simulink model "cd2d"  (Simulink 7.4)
settings: Solver=ode45  StartTime=0.0  StopTime=10.0  RelTol=1e-3
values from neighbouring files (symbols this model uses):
  B = 8    [cd2d_par.m]
  D = 5    [cd2d_par.m]
  T = 12    [cd2d_par.m]
libraries: simulink x2

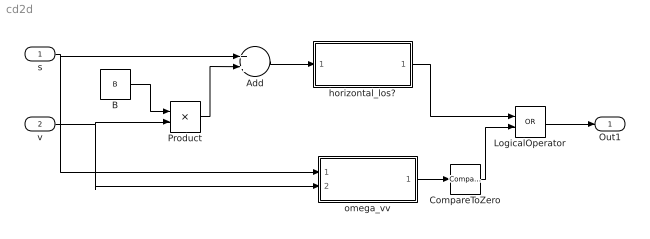
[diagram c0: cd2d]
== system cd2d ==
  s : Inport  Description=|  OutDataType=fixdt(1, 16)  OutScaling=2^0
      | begin dimension                   
      | output _ : [(length kilometer 1)];
      | end dimension
  v : Inport  Description=|  Port=2  OutDataType=fixdt(1, 16)  OutScaling=2^0
      | begin dimension                                 
      | output _ : [(length kilometer 1, time hour -1)];
      | end dimension
  Add : Sum  OutDataType=fixdt(1, 16)  OutScaling=2^-10
  B : Constant  Description=|  Value=B  OutDataType=fixdt(1, 16)  OutScaling=2^0
      | begin dimension            
      | output _ : [(time hour 1)];
      | end dimension
  CompareToZero : simulink/Logic and Bit Operations/Compare To Zero  SystemSampleTime=-1  relop=<  LogicOutDataTypeMode=uint8
  LogicalOperator : Logic  Operator=OR  AllPortsSameDT=off  OutDataTypeMode=boolean  LogicDataType=fixdt(0, 8)  OutDataTypeStr=boolean
  Product : Product  OutDataType=fixdt(1, 16)  OutScaling=2^0
  horizontal_los? : Subsystem
  omega_vv : Subsystem
  Out1 : Outport  Description=|  OutDataType=fixdt(1, 16)  OutScaling=2^0
      | begin dimension             
      | input _ : [(dimensionless)];
      | end dimension
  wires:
  s/1 -> Add/1, omega_vv/1(s)
  B/1 -> Product/1
  v/1 -> Product/2, omega_vv/2(v)
  Product/1 -> Add/2
  Add/1 -> horizontal_los?/1(In1)
  horizontal_los?/1(Out1) -> LogicalOperator/1
  omega_vv/1(Out1) -> CompareToZero/1
  CompareToZero/1 -> LogicalOperator/2
  LogicalOperator/1 -> Out1/1

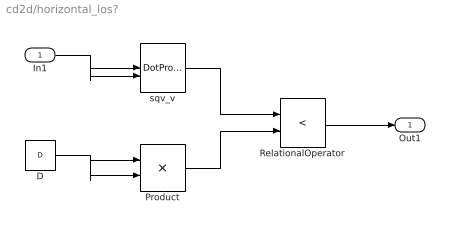
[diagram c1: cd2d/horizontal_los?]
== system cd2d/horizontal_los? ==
  In1 : Inport  Description=|  OutDataType=fixdt(1, 16)  OutScaling=2^0
      | begin dimension                   
      | output _ : [(length kilometer 1)];
      | end dimension
  D : Constant  Description=|  Value=D  OutDataType=fixdt(1, 16)  OutScaling=2^0
      | begin dimension                   
      | output _ : [(length kilometer 1)];
      | end dimension
  Product : Product  OutDataType=fixdt(1, 16)  OutScaling=2^0
  RelationalOperator : RelationalOperator  Operator=<  LogicOutDataTypeMode=boolean  LogicDataType=fixdt(0, 8)  OutDataTypeStr=boolean
  sqv_v : DotProduct  OutDataType=fixdt(1, 16)  OutScaling=2^-10
  Out1 : Outport  Description=|  OutDataType=fixdt(1, 16)  OutScaling=2^0
      | begin dimension             
      | input _ : [(dimensionless)];
      | end dimension
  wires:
  In1/1 -> sqv_v/1, sqv_v/2
  sqv_v/1 -> RelationalOperator/1
  Product/1 -> RelationalOperator/2
  RelationalOperator/1 -> Out1/1
  D/1 -> Product/1, Product/2

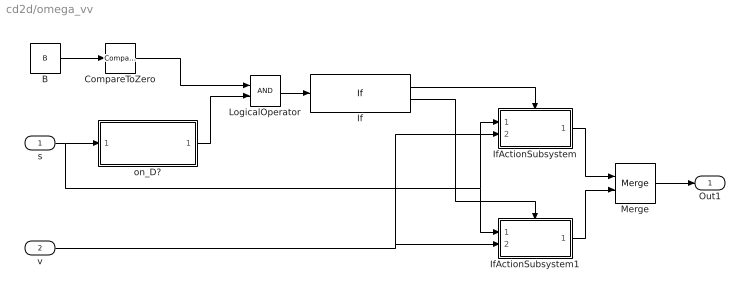
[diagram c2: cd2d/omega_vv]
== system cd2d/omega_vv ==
  s : Inport  Description=|  OutDataType=fixdt(1, 16)  OutScaling=2^0
      | begin dimension                   
      | output _ : [(length kilometer 1)];
      | end dimension
  v : Inport  Description=|  Port=2  OutDataType=fixdt(1, 16)  OutScaling=2^0
      | begin dimension                                 
      | output _ : [(length kilometer 1, time hour -1)];
      | end dimension
  B : Constant  Description=|  Value=B  OutDataType=fixdt(1, 16)  OutScaling=2^0
      | begin dimension            
      | output _ : [(time hour 1)];
      | end dimension
  CompareToZero : simulink/Logic and Bit Operations/Compare To Zero  SystemSampleTime=-1  relop===  LogicOutDataTypeMode=uint8
  If : If  IfExpression=u1
  IfActionSubsystem : Subsystem  TreatAsAtomicUnit=on
  IfActionSubsystem1 : Subsystem  TreatAsAtomicUnit=on
  LogicalOperator : Logic  AllPortsSameDT=off  OutDataTypeMode=boolean  LogicDataType=fixdt(0, 8)  OutDataTypeStr=boolean
  Merge : Merge
  on_D? : Subsystem
  Out1 : Outport  OutDataType=fixdt(1, 16)  OutScaling=2^0
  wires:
  s/1 -> IfActionSubsystem/1(s), IfActionSubsystem1/1(s), on_D?/1(In1)
  B/1 -> CompareToZero/1
  CompareToZero/1 -> LogicalOperator/1
  on_D?/1(Out1) -> LogicalOperator/2
  LogicalOperator/1 -> If/1
  Merge/1 -> Out1/1
  IfActionSubsystem/1(Out1) -> Merge/1
  IfActionSubsystem1/1(Out1) -> Merge/2
  If/2 -> IfActionSubsystem1/Action
  If/1 -> IfActionSubsystem/Action
  v/1 -> IfActionSubsystem/2(v), IfActionSubsystem1/2(v)

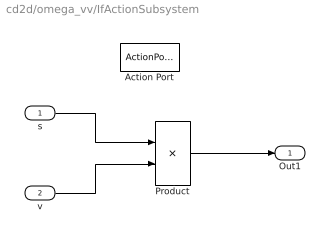
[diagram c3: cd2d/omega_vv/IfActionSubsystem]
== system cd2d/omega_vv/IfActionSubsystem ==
  s : Inport  Description=|  OutDataType=fixdt(1, 16)  OutScaling=2^0
      | begin dimension                   
      | output _ : [(length kilometer 1)];
      | end dimension
  v : Inport  Description=|  Port=2  OutDataType=fixdt(1, 16)  OutScaling=2^0
      | begin dimension                                 
      | output _ : [(length kilometer 1, time hour -1)];
      | end dimension
  Action Port : ActionPort  ActionType=then
  Product : Product  OutDataType=fixdt(1, 16)  OutScaling=2^0
  Out1 : Outport  Description=|  OutDataType=fixdt(1, 16)  OutScaling=2^0
      | begin dimension                                
      | input _ : [(length kilometer 2, time hour -1)];
      | end dimension
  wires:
  Product/1 -> Out1/1
  s/1 -> Product/1
  v/1 -> Product/2

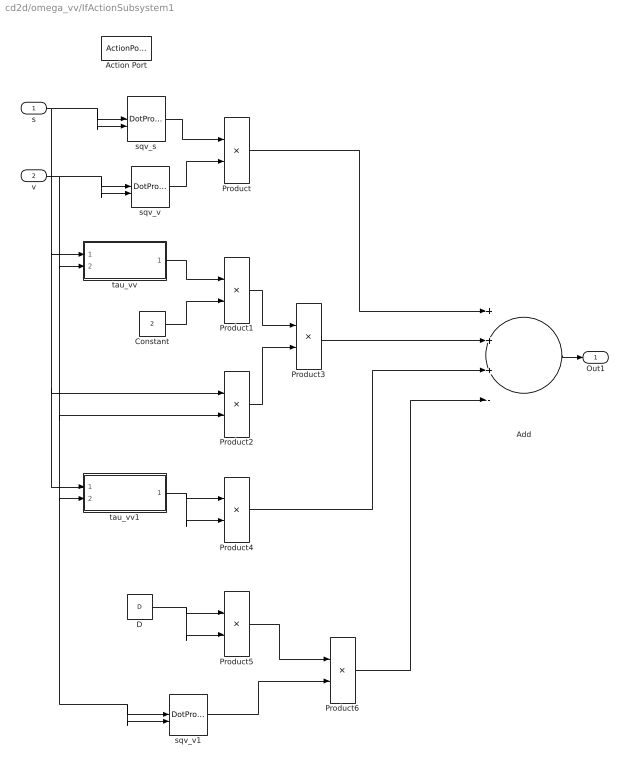
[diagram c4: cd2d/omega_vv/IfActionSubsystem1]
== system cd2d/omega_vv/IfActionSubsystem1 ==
  s : Inport  Description=|  OutDataType=fixdt(1, 16)  OutScaling=2^0
      | begin dimension                   
      | output _ : [(length kilometer 1)];
      | end dimension
  v : Inport  Description=|  Port=2  OutDataType=fixdt(1, 16)  OutScaling=2^0
      | begin dimension                                 
      | output _ : [(length kilometer 1, time hour -1)];
      | end dimension
  Action Port : ActionPort  ActionType=else
  Add : Sum  Inputs=+++-  OutDataType=fixdt(1, 16)  OutScaling=2^-10
  Constant : Constant  Description=|  Value=2  OutDataType=fixdt(1, 16)  OutScaling=2^0
      | begin dimension              
      | output _ : [(dimensionless)];
      | end dimension
  D : Constant  Description=|  Value=D  OutDataType=fixdt(1, 16)  OutScaling=2^0
      | begin dimension                   
      | output _ : [(length kilometer 1)];
      | end dimension
  Product{,1..6} (7 alike) : Product  OutDataType=fixdt(1, 16)  OutScaling=2^0
  sqv_s : DotProduct  OutDataType=fixdt(1, 16)  OutScaling=2^-10
  sqv_v : DotProduct  OutDataType=fixdt(1, 16)  OutScaling=2^-10
  sqv_v1 : DotProduct  OutDataType=fixdt(1, 16)  OutScaling=2^-10
  tau_vv : Subsystem
  tau_vv1 : Subsystem
  Out1 : Outport  Description=|  OutDataType=fixdt(1, 16)  OutScaling=2^0
      | begin dimension                                
      | input _ : [(length kilometer 4, time hour -2)];
      | end dimension
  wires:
  s/1 -> Product2/1, tau_vv1/1(s), tau_vv/1(s), sqv_s/1, sqv_s/2
  v/1 -> Product2/2, sqv_v1/1, sqv_v1/2, tau_vv1/2(v), tau_vv/2(v), sqv_v/1, sqv_v/2
  sqv_s/1 -> Product/1
  sqv_v/1 -> Product/2
  Product/1 -> Add/1
  Add/1 -> Out1/1
  tau_vv/1(Out1) -> Product1/1
  Constant/1 -> Product1/2
  Product1/1 -> Product3/1
  Product2/1 -> Product3/2
  Product3/1 -> Add/2
  tau_vv1/1(Out1) -> Product4/1, Product4/2
  Product4/1 -> Add/3
  D/1 -> Product5/1, Product5/2
  Product5/1 -> Product6/1
  sqv_v1/1 -> Product6/2
  Product6/1 -> Add/4

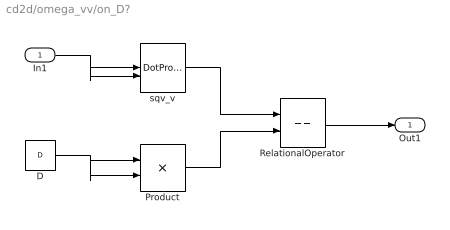
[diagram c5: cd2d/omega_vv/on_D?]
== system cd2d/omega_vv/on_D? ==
  In1 : Inport  Description=|  OutDataType=fixdt(1, 16)  OutScaling=2^0
      | begin dimension                   
      | output _ : [(length kilometer 1)];
      | end dimension
  D : Constant  Description=|  Value=D  OutDataType=fixdt(1, 16)  OutScaling=2^0
      | begin dimension                   
      | output _ : [(length kilometer 1)];
      | end dimension
  Product : Product  OutDataType=fixdt(1, 16)  OutScaling=2^0
  RelationalOperator : RelationalOperator  Operator===  LogicOutDataTypeMode=boolean  LogicDataType=fixdt(0, 8)  OutDataTypeStr=boolean
  sqv_v : DotProduct  OutDataType=fixdt(1, 16)  OutScaling=2^-10
  Out1 : Outport  Description=|  OutDataType=fixdt(1, 16)  OutScaling=2^0
      | begin dimension             
      | input _ : [(dimensionless)];
      | end dimension
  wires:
  In1/1 -> sqv_v/1, sqv_v/2
  sqv_v/1 -> RelationalOperator/1
  Product/1 -> RelationalOperator/2
  RelationalOperator/1 -> Out1/1
  D/1 -> Product/1, Product/2

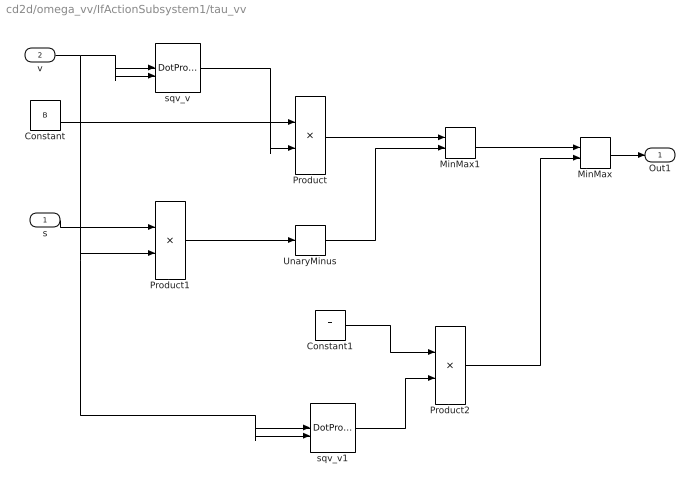
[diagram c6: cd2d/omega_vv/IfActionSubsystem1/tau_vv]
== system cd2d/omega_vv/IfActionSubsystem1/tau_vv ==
  s : Inport  Description=|  OutDataType=fixdt(1, 16)  OutScaling=2^0
      | begin dimension                   
      | output _ : [(length kilometer 1)];
      | end dimension
  v : Inport  Description=|  Port=2  OutDataType=fixdt(1, 16)  OutScaling=2^0
      | begin dimension                                 
      | output _ : [(length kilometer 1, time hour -1)];
      | end dimension
  Constant : Constant  Description=|  Value=B  OutDataType=fixdt(1, 16)  OutScaling=2^0
      | begin dimension            
      | output _ : [(time hour 1)];
      | end dimension
  Constant1 : Constant  Description=|  Value=T  OutDataType=fixdt(1, 16)  OutScaling=2^0
      | begin dimension            
      | output _ : [(time hour 1)];
      | end dimension
  MinMax : MinMax  Inputs=2  OutDataType=fixdt(1, 16)  OutScaling=2^0
  MinMax1 : MinMax  Function=max  Inputs=2  OutDataType=fixdt(1, 16)  OutScaling=2^0
  Product : Product  OutDataType=fixdt(1, 16)  OutScaling=2^0
  Product1 : Product  OutDataType=fixdt(1, 16)  OutScaling=2^0
  Product2 : Product  OutDataType=fixdt(1, 16)  OutScaling=2^0
  UnaryMinus : UnaryMinus
  sqv_v : DotProduct  OutDataType=fixdt(1, 16)  OutScaling=2^-10
  sqv_v1 : DotProduct  OutDataType=fixdt(1, 16)  OutScaling=2^-10
  Out1 : Outport  Description=|  OutDataType=fixdt(1, 16)  OutScaling=2^0
      | begin dimension                                
      | input _ : [(length kilometer 2, time hour -1)];
      | end dimension
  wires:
  MinMax1/1 -> MinMax/1
  v/1 -> Product1/2, sqv_v1/1, sqv_v1/2, sqv_v/1, sqv_v/2
  Constant/1 -> Product/1
  sqv_v/1 -> Product/2
  Product/1 -> MinMax1/1
  Product1/1 -> UnaryMinus/1
  UnaryMinus/1 -> MinMax1/2
  s/1 -> Product1/1
  Constant1/1 -> Product2/1
  sqv_v1/1 -> Product2/2
  Product2/1 -> MinMax/2
  MinMax/1 -> Out1/1

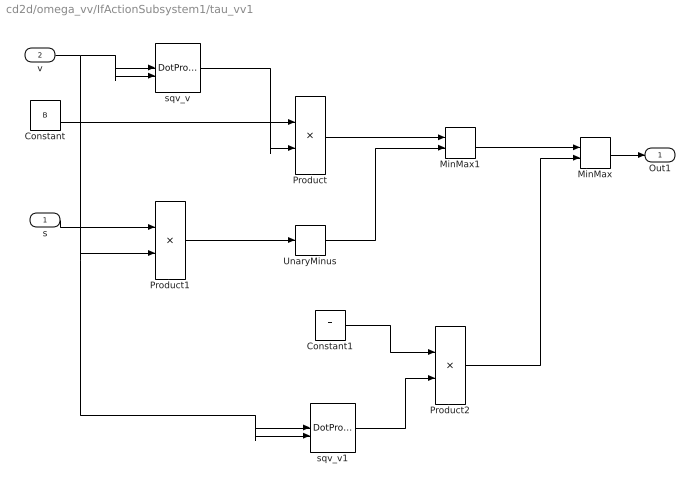
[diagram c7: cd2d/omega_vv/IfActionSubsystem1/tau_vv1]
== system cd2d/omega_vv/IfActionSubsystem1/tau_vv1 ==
  s : Inport  Description=|  OutDataType=fixdt(1, 16)  OutScaling=2^0
      | begin dimension                   
      | output _ : [(length kilometer 1)];
      | end dimension
  v : Inport  Description=|  Port=2  OutDataType=fixdt(1, 16)  OutScaling=2^0
      | begin dimension                                 
      | output _ : [(length kilometer 1, time hour -1)];
      | end dimension
  Constant : Constant  Description=|  Value=B  OutDataType=fixdt(1, 16)  OutScaling=2^0
      | begin dimension            
      | output _ : [(time hour 1)];
      | end dimension
  Constant1 : Constant  Description=|  Value=T  OutDataType=fixdt(1, 16)  OutScaling=2^0
      | begin dimension            
      | output _ : [(time hour 1)];
      | end dimension
  MinMax : MinMax  Inputs=2  OutDataType=fixdt(1, 16)  OutScaling=2^0
  MinMax1 : MinMax  Function=max  Inputs=2  OutDataType=fixdt(1, 16)  OutScaling=2^0
  Product : Product  OutDataType=fixdt(1, 16)  OutScaling=2^0
  Product1 : Product  OutDataType=fixdt(1, 16)  OutScaling=2^0
  Product2 : Product  OutDataType=fixdt(1, 16)  OutScaling=2^0
  UnaryMinus : UnaryMinus
  sqv_v : DotProduct  OutDataType=fixdt(1, 16)  OutScaling=2^-10
  sqv_v1 : DotProduct  OutDataType=fixdt(1, 16)  OutScaling=2^-10
  Out1 : Outport  Description=|  OutDataType=fixdt(1, 16)  OutScaling=2^0
      | begin dimension                                
      | input _ : [(length kilometer 2, time hour -1)];
      | end dimension
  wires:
  MinMax1/1 -> MinMax/1
  v/1 -> Product1/2, sqv_v1/1, sqv_v1/2, sqv_v/1, sqv_v/2
  Constant/1 -> Product/1
  sqv_v/1 -> Product/2
  Product/1 -> MinMax1/1
  Product1/1 -> UnaryMinus/1
  UnaryMinus/1 -> MinMax1/2
  s/1 -> Product1/1
  Constant1/1 -> Product2/1
  sqv_v1/1 -> Product2/2
  Product2/1 -> MinMax/2
  MinMax/1 -> Out1/1
